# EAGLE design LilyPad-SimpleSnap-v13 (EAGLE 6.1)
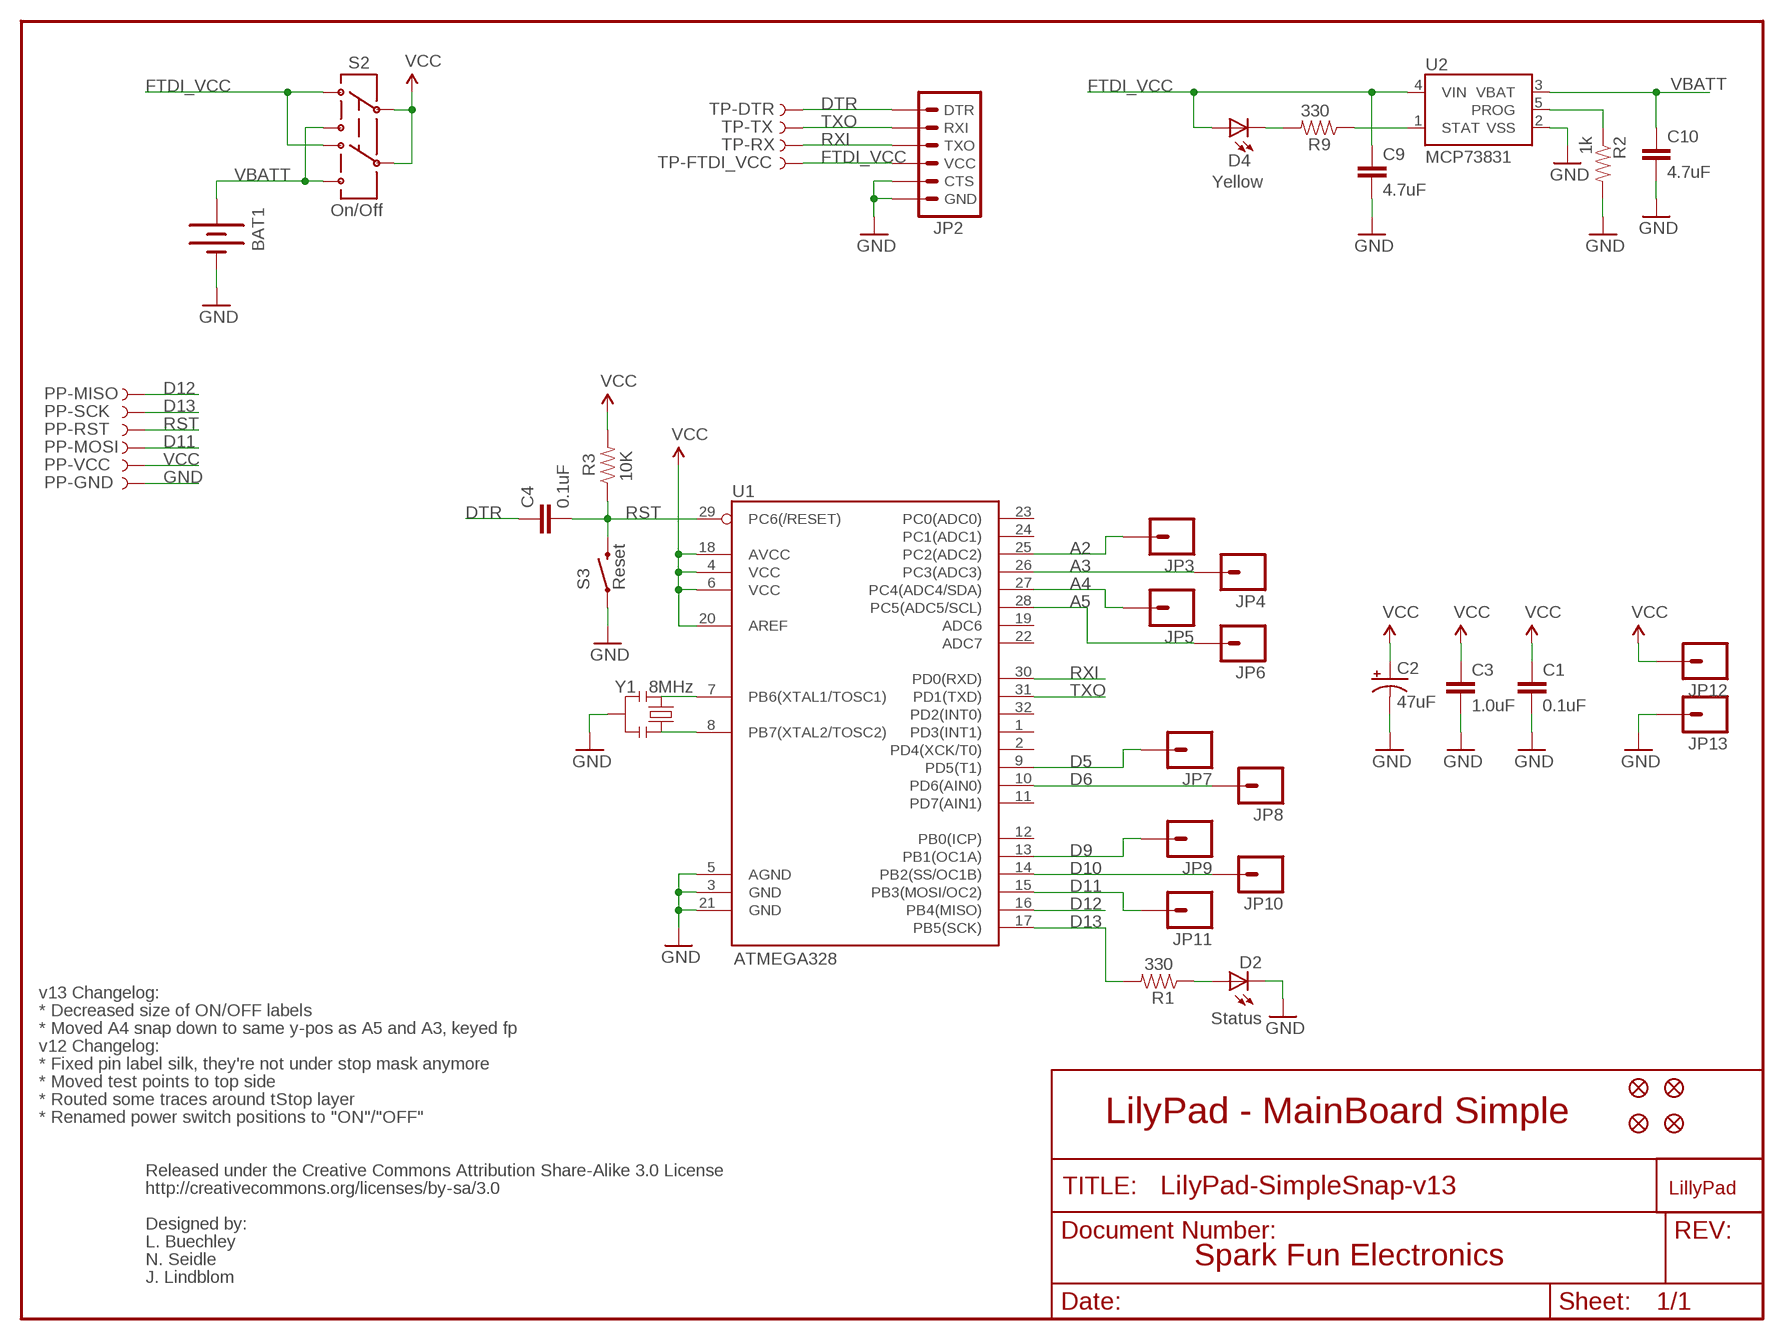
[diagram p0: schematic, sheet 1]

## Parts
BAT1  BATTERY110-TABS  [LIPO-110-TABS]
C1  0.1uF  CAP0402-CAP  [0402-CAP]
C2  47uF  CAP_POL3528  [EIA3528]
C3  1.0uF  CAP0402-CAP  [0402-CAP]
C4  0.1uF  CAP0402-CAP  [0402-CAP]
C9  4.7uF  CAP0402-CAP  [0402-CAP]
C10  4.7uF  CAP0402-CAP  [0402-CAP]
D2  Status  LED0603  [LED-0603]
D4  Yellow  LED0603  [LED-0603]
JP1  FIDUCIALUFIDUCIAL  [MICRO-FIDUCIAL]
JP2  ARDUINO_SERIAL_PROGRAMSMD  [1X06-SMD]
JP3  M01SNAP-FEMALE_LARGE  M01SNAP-FEMALE  [SNAP-FEMALE]
JP4  M01SNAP-FEMALE_LARGE  M01SNAP-FEMALE  [SNAP-FEMALE]
JP5  M01SNAP-FEMALE_LARGE  M01SNAP-FEMALE  [SNAP-FEMALE]
JP6  M01SNAP-FEMALE_LARGE  M01SNAP-FEMALE  [SNAP-FEMALE]
JP7  M01SNAP-FEMALE_LARGE  M01SNAP-FEMALE  [SNAP-FEMALE]
JP8  M01SNAP-FEMALE_LARGE  M01SNAP-FEMALE  [SNAP-FEMALE]
JP9  M01SNAP-FEMALE_LARGE  M01SNAP-FEMALE  [SNAP-FEMALE]
JP10  M01SNAP-FEMALE_LARGE  M01SNAP-FEMALE  [SNAP-FEMALE]
JP11  M01SNAP-FEMALE_LARGE  M01SNAP-FEMALE  [SNAP-FEMALE]
JP12  M01SNAP-FEMALE_LARGE  M01SNAP-FEMALE  [SNAP-FEMALE]
JP13  M01SNAP-FEMALE_LARGE  M01SNAP-FEMALE  [SNAP-FEMALE]
JP14  FIDUCIALUFIDUCIAL  [MICRO-FIDUCIAL]
JP15  FIDUCIALUFIDUCIAL  [MICRO-FIDUCIAL]
JP16  FIDUCIALUFIDUCIAL  [MICRO-FIDUCIAL]
PP-GND  TEST-POINT3X5  [PAD.03X.05]
PP-MISO  TEST-POINT3X5  [PAD.03X.05]
PP-MOSI  TEST-POINT3X5  [PAD.03X.05]
PP-RST  TEST-POINT3X5  [PAD.03X.05]
PP-SCK  TEST-POINT3X5  [PAD.03X.05]
PP-VCC  TEST-POINT3X5  [PAD.03X.05]
R1  330  RESISTOR0402-RES  [0402-RES]
R2  1k  RESISTOR0402-RES  [0402-RES]
R3  10K  RESISTOR0402-RES  [0402-RES]
R9  330  RESISTOR0402-RES  [0402-RES]
S2  On/Off  AYZ0202  [AYZ0202]
S3  Reset  SWITCH-MOMENTARY-2SMD  [TACTILE_SWITCH_SMD]
TP-DTR  TEST-POINT3X5  [PAD.03X.05]
TP-FTDI_VCC  TEST-POINT3X5  [PAD.03X.05]
TP-RX  TEST-POINT3X5  [PAD.03X.05]
TP-TX  TEST-POINT3X5  [PAD.03X.05]
U1  ATMEGA328  ATMEGA168  [TQFP32-08]
U2  MCP73831  [SOT23-5]
U$2  LOGO-LPLP  [LOGO-LILYPAD]
Y1  8MHz  RESONATORSMD  [RESONATOR-SMD]

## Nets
A2: JP3.1 U1.25(PC2(ADC2))
A3: JP4.1 U1.26(PC3(ADC3))
A4: JP5.1 U1.27(PC4(ADC4/SDA))
A5: JP6.1 U1.28(PC5(ADC5/SCL))
D5: JP7.1 U1.9(PD5(T1))
D6: JP8.1 U1.10(PD6(AIN0))
D9: JP9.1 U1.13(PB1(OC1A))
D10: JP10.1 U1.14(PB2(SS/OC1B))
D11: JP11.1 PP-MOSI.P$1 U1.15(PB3(MOSI/OC2))
D12: PP-MISO.P$1 U1.16(PB4(MISO))
D13: PP-SCK.P$1 R1.2 U1.17(PB5(SCK))
DTR: C4.1 JP2.1(DTR) TP-DTR.P$1
FTDI_VCC: C9.1 D4.A JP2.4(VCC) S2.3 S2.6 TP-FTDI_VCC.P$1 U2.4(VIN)
GND [VCC]: BAT1.- C1.2 C2.C(-) C3.2 C9.2 C10.2 D2.C JP2.5(CTS) JP2.6(GND) JP13.1 PP-GND.P$1 R2.2 S3.1 U1.3(GND) U1.5(AGND) U1.21(GND) U2.2(VSS) Y1.2
N$1: U1.7(PB6(XTAL1/TOSC1)) Y1.1
N$2: D2.A R1.1
N$3: U1.8(PB7(XTAL2/TOSC2)) Y1.3
N$8: D4.C R9.2
PROG: R2.1 U2.5(PROG)
RST: C4.2 PP-RST.P$1 R3.1 S3.3 U1.29(PC6(/RESET))
RXI: JP2.3(TXO) TP-RX.P$1 U1.30(PD0(RXD))
STAT: R9.1 U2.1(STAT)
TXO: JP2.2(RXI) TP-TX.P$1 U1.31(PD1(TXD))
VBATT: BAT1.+ C10.1 S2.1 S2.4 U2.3(VBAT)
VCC [VCC]: C1.1 C2.A(+) C3.1 JP12.1 PP-VCC.P$1 R3.2 S2.2 S2.5 U1.4(VCC) U1.6(VCC) U1.18(AVCC) U1.20(AREF)
Unconnected: U1.1(PD3(INT1)) U1.2(PD4(XCK/T0)) U1.11(PD7(AIN1)) U1.12(PB0(ICP)) U1.19(ADC6) U1.22(ADC7) U1.23(PC0(ADC0)) U1.24(PC1(ADC1)) U1.32(PD2(INT0))

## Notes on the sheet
- v13 Changelog:
- * Decreased size of ON/OFF labels
- * Moved A4 snap down to same y-pos as A5 and A3, keyed fp
- v12 Changelog:
- * Fixed pin label silk, they're not under stop mask anymore
- * Moved test points to top side
- * Routed some traces around tStop layer
- * Renamed power switch positions to "ON"/"OFF" | LilyPad - MainBoard Simple
- Released under the Creative Commons Attribution Share-Alike 3.0 License
- http://creativecommons.org/licenses/by-sa/3.0
- Designed by:
- L. Buechley
- N. Seidle | Spark Fun Electronics
- J. Lindblom

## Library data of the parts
BAT1 = SparkFun:BATTERY: Battery Holders
C1 C3 C4 C9 C10 = SparkFun:CAP: Capacitor
C2 = SparkFun:CAP_POL: Capacitor Polarized
D2 D4 = SparkFun:LED: LEDs
JP1 JP14-JP16 = SparkFun:FIDUCIAL: Fiducial Alignment Points
JP2 = SparkFun:ARDUINO_SERIAL_PROGRAM
JP3-JP13 = SparkFun:M01: Header 1
PP-GND PP-MISO PP-MOSI PP-RST PP-SCK PP-VCC TP-DTR TP-FTDI_VCC TP-RX TP-TX = SparkFun:TEST-POINT
R1-R3 R9 = SparkFun:RESISTOR: Resistor
S2 = SparkFun:AYZ0202: SPDT Slide Switch Simple SMD single-pull double-throw slide switch. Good for less than 350mA power switch, switching UARTs between devices, etc. Spark Fun Electronics SKU : COM-00597
S3 = SparkFun:SWITCH-MOMENTARY-2
U1 = SparkFun:ATMEGA168
U2 = SparkFun:MCP73831: Microchip's MCP73831 Miniature single cell, fully integrated Li-Ion, Li-polymer charge management controller http://ww1.microchip.com/downloads/en/DeviceDoc/21984a.pdf
U$2 = LilyPad-Wearables:LOGO-LP
Y1 = SparkFun:RESONATOR: Resonator Small SMD resonator. This is the itty bitty 10/20MHz resonators with built in caps. CSTCE10M0G55 and CSTCE20M0V53. Footprint has been reviewed closely but hasn't been tested yet.

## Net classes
0 Default: width 0.203 mm
1 VCC: width 0.254 mm

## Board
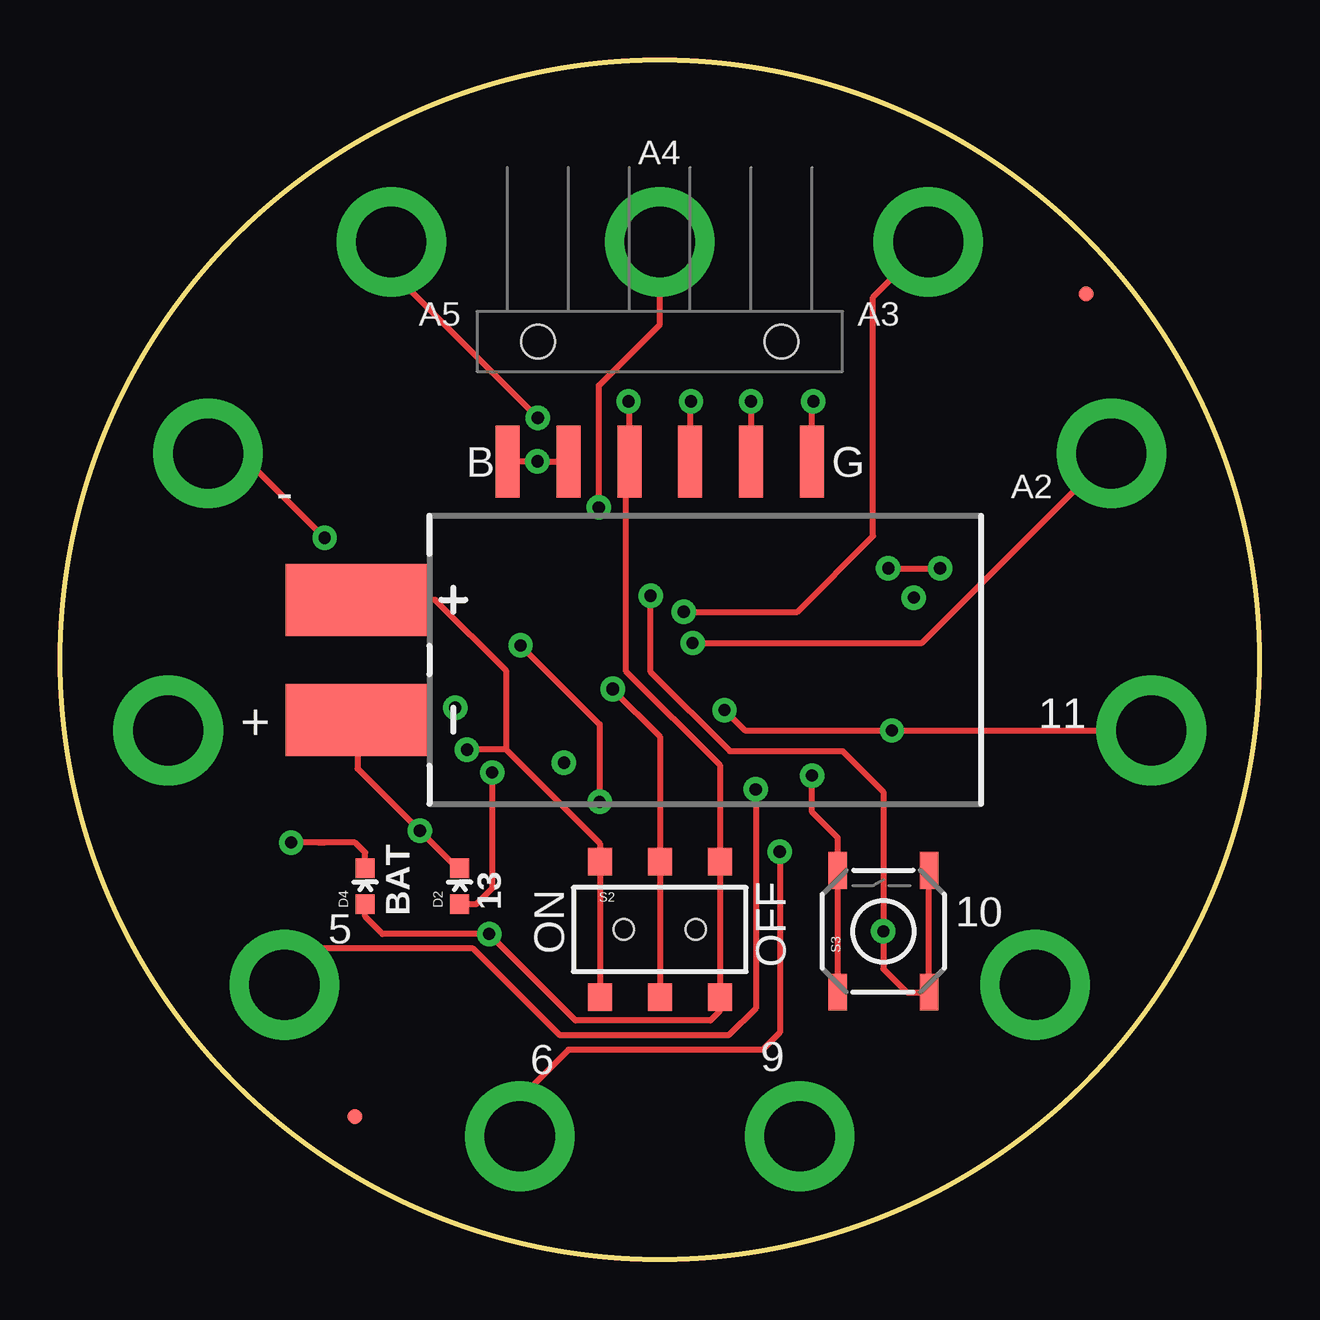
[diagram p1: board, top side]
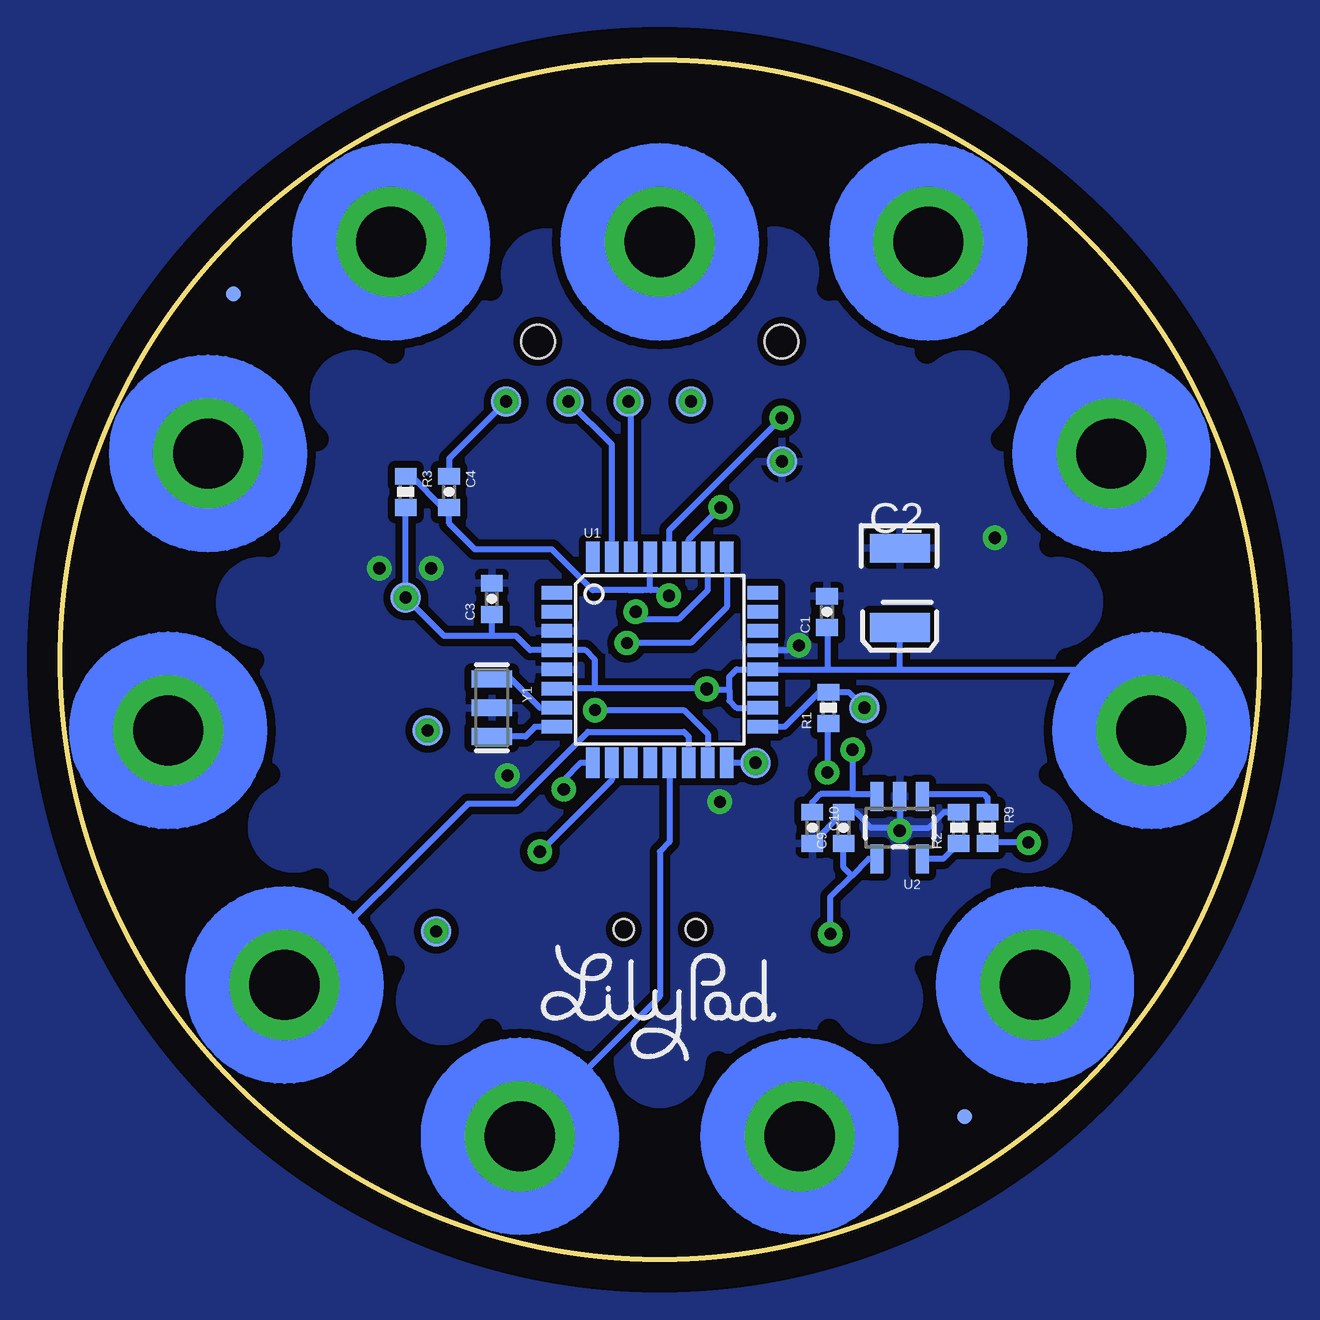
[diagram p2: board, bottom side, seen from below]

Size 50 x 50 mm. Coordinates in mm from the lower left corner, seen from the top.
Outline: circle at 25,25 radius 25
Copper layers (1*16): Top 0.035mm / dielectric 1.5mm / Bottom 0.035mm
Design rules: minimum track width 8mil, minimum drill 20mil, track to track 8mil, track to pad 8mil, pad to pad 8mil, via to via 8mil, smd to smd 8mil, copper to edge 8mil, drill to drill 8mil, minimum pad ring 12mil, minimum via ring 10mil, stop-mask expansion 4mil, vias tented up to drill 20mil, thermal gap 10mil
bRestrict: area 2.4,2.4 to 47.6,47.6; area 21,42.8 to 23.5,44; area 31.6,41.3 to 34.4,43; area 36.3,38.4 to 38.9,40.7; area 40,34.1 to 42,36.9; area 42.2,29.2 to 43.6,31.8; area 42.8,23.9 to 44,26.2; area 42.2,18.2 to 43.7,20.9; area 36.3,9.4 to 39,11.7; area 31.7,7 to 34.5,8.7; area 26.5,6 to 28.9,7.3; area 21.1,6 to 23.6,7.3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; 22 lines

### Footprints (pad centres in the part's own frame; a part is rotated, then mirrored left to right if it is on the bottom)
LIPO-110-TABS = smd 3 x 6: + 2.5,14.5; - -2.5,14.5
0402-CAP = smd 0.7 x 0.9: 1 -0.65,0; 2 0.65,0
EIA3528 = smd 1.2 x 2.5: A 1.65,0; C -1.65,0
LED-0603 = smd 0.8 x 0.8: A 0,-0.75; C 0,0.75
MICRO-FIDUCIAL = smd 0.635 x 0.635: 1 0,0
1X06-SMD = smd 1 x 3: 1 -6.35,5; 2 -3.81,5; 3 -1.27,5; 4 1.27,5; 5 3.81,5; 6 6.35,5 | hole 1.4: -5.08,0; 5.08,0
SNAP-FEMALE = drill 2.921 pad 4.572: 1 0,0
PAD.03X.05 = smd 1.27 x 1.27: P$1 0,0
0402-RES = smd 0.7 x 0.9: 1 -0.65,0; 2 0.65,0
AYZ0202 = smd 1 x 1.15: 1 -2.5,2.825; 2 0,2.825; 3 2.5,2.825; 4 -2.5,-2.825; 5 0,-2.825; 6 2.5,-2.825 | hole 0.85: 1.5,0; -1.5,0
TACTILE_SWITCH_SMD = smd 1.524 x 0.762: 1 -2.54,1.905; 2 2.54,1.905; 3 -2.54,-1.905; 4 2.54,-1.905
TQFP32-08 = smd 1.27 x 0.559: 1 -4.293,2.8; 2 -4.293,2; 3 -4.293,1.2; 4 -4.293,0.4; 5 -4.293,-0.4; 6 -4.293,-1.2; 7 -4.293,-2; 8 -4.293,-2.8; 17 4.293,-2.8; 18 4.293,-2; 19 4.293,-1.2; 20 4.293,-0.4; 21 4.293,0.4; 22 4.293,1.2; 23 4.293,2; 24 4.293,2.8 | smd 0.559 x 1.27: 9 -2.8,-4.293; 10 -2,-4.293; 11 -1.2,-4.293; 12 -0.4,-4.293; 13 0.4,-4.293; 14 1.2,-4.293; 15 2,-4.293; 16 2.8,-4.293; 25 2.8,4.293; 26 2,4.293; 27 1.2,4.293; 28 0.4,4.293; 29 -0.4,4.293; 30 -1.2,4.293; 31 -2,4.293; 32 -2.8,4.293
SOT23-5 = smd 0.55 x 1.2: 1 -0.95,-1.3; 2 0,-1.3; 3 0.95,-1.3; 4 0.95,1.3; 5 -0.95,1.3
RESONATOR-SMD = smd 0.7 x 1.7: 1 -1.2,0; 2 0,0; 3 1.2,0

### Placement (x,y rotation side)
BAT1  26.91,25 90 top
C1  18.03,27 90 bottom
C2  15,28 270 bottom
C3  32,27.54 90 bottom
C4  33.78,32 270 bottom
C9  17.34,18 90 bottom
C10  18.64,18 270 bottom
D2  16.66,15.56 0 top
D4  12.72,15.56 0 top
JP1  42.78,40.24 0 top
JP2  25,38.27 180 top
JP3  43.83,33.6 0 bottom
JP4  36.19,42.41 0 bottom
JP5  25,42.41 0 bottom
JP6  13.81,42.41 0 bottom
JP7  9.36,11.44 0 bottom
JP8  19.17,5.14 0 bottom
JP9  30.83,5.14 0 bottom
JP10  40.64,11.44 0 bottom
JP11  45.49,22.05 0 bottom
JP12  4.51,22.05 0 bottom
JP13  6.17,33.6 0 bottom
JP14  12.3,5.95 0 top
JP15  12.3,5.95 0 bottom
JP16  42.78,40.24 0 bottom
PP-GND  19.9,33.27 0 bottom
PP-MISO  21.01,20.71 180 bottom
PP-MOSI  34.68,22.05 0 bottom
PP-RST  34.32,13.68 0 bottom
PP-SCK  16.47,23 180 bottom
PP-VCC  35.59,27.59 0 bottom
R1  17.97,23 90 bottom
R2  12.54,18 90 bottom
R3  35.59,32 270 bottom
R9  11.34,18 270 bottom
S2  25,13.76 0 top
S3  34.32,13.68 90 top
TP-DTR  31.4,35.77 0 bottom
TP-FTDI_VCC  23.7,35.77 0 bottom
TP-RX  26.3,35.77 0 bottom
TP-TX  28.8,35.77 90 bottom
U1  25,25 0 bottom
U2  15,18 180 bottom
U$2  25,11.03 0 bottom
Y1  32,23 270 bottom

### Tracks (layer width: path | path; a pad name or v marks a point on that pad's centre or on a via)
A2  (via drill 0.51)
  Top 0.254: JP3.1 35.93,25.7 v26.37,25.7
  Bottom 0.254: v26.37,25.7 23.7,25.7 22.2,27.2 U1.25
A3  (via drill 0.51)
  Top 0.254: v26,27 30.73,27 33.89,30.16 33.89,40.11 JP4.1
  Bottom 0.254: U1.26 23,27.9 24.2,26.7 25.7,26.7 v26,27
A4  (via drill 0.51)
  Top 0.254: v22.46,31.35 22.46,36.43 25,38.97 JP5.1
  Bottom 0.254: U1.27 23.8,30.01 v22.46,31.35
A5  (via drill 0.51)
  Top 0.254: v19.92,35.08 13.81,41.19 JP6.1
  Bottom 0.254: U1.28 24.6,30.4 v19.92,35.08
D5  (via drill 0.51)
  Top 0.254: v29,19.6 29,10.48 27.87,9.35 20.84,9.35 17.23,12.96 10.87,12.96 JP7.1
  Bottom 0.254: U1.9 28.29,20.71 29,20 v29,19.6
D6  (via drill 0.51)
  Top 0.254: v30,17 30,9.46 29.28,8.74 21.19,8.74 19.17,6.72 JP8.1
  Bottom 0.254: U1.10 27,20 v30,17
D9
  Bottom 0.254: U1.13 24.6,17.4 25,17 25,10.97 JP9.1
D10
  Bottom 0.254: U1.14 23.8,21.8 24,22 28,22 31,19 33,19 40.56,11.44 JP10.1
D11  (via drill 0.51)
  Top 0.254: v27.7,22.9 28.55,22.05 PP-MOSI.P$1 JP11.1
  Bottom 0.254: U1.15 23,21.9 24,22.9 v27.7,22.9
  other vias: 34.68,22.05
D12  (via drill 0.51)
  Bottom 0.254: PP-MISO.P$1 U1.16
  other vias: 21.01,20.71
D13  (via drill 0.51)
  Bottom 0.254: U1.17 19.8,22.2 18.35,23.65 R1.2 17.12,23.65 PP-SCK.P$1
  other vias: 16.47,23
DTR  (via drill 0.51)
  Top 0.254: JP2.1 31.35,35.72 TP-DTR.P$1
  Bottom 0.254: C4.1 33.78,33.39 TP-DTR.P$1
  other vias: 31.4,35.77
FTDI_VCC  (via drill 0.51)
  Top 0.254: 23.73,33 JP2.4 | 23.73,33 23.6,32.87 23.6,24.51 27.5,20.61 S2.3 S2.6 27.5,10.36 27.11,9.97 21.49,9.97 v17.89,13.57 13.44,13.57 12.72,14.29 D4.A | 23.73,33 23.73,35.74 TP-FTDI_VCC.P$1
  Bottom 0.254: U2.4 16.3,16.7 17,16 | C9.1 17.34,16.34 17,16 | v17.89,13.57 17.89,15.11 17,16
  other vias: 23.7,35.77
GND  (via drill 0.51)
  Top 0.254: JP2.6 PP-GND.P$1 JP2.5 | v34.52,28.81 v36.68,28.81 | v31.35,20.17 31.35,18.65 32.41,17.59 S3.1 | D2.C 16.56,16.31 v15,17.87 12.4,20.47 BAT1.- | JP13.1 7.51,33.6 v11.03,30.08 | v22.49,19.08 22.49,22.31 v19.2,25.6
  Bottom 0.254: R2.2 13.15,18.65 13.8,18 14.97,18 | C10.2 C9.2 16.85,18.65 16.2,18 14.97,18 | v19.2,25.6 19.4,25.4 U1.21 | U2.2 15,18.03 14.97,18
  other vias: 19.9,33.27
  pour Bottom (isolate 0.305): -3.54,53.54 53.54,53.54 53.54,-3.54 -3.54,-3.54
N$1
  Bottom 0.254: U1.7 30,23 31.2,24.2 Y1.1
N$2  (via drill 0.51)
  Top 0.254: D2.A 17.35,14.81 18.02,15.47 v18.02,20.3
  Bottom 0.254: v18.02,20.3 18.02,22.3 R1.1
N$3
  Bottom 0.254: U1.8 30.2,22.2 30.6,21.8 Y1.3
N$8  (via drill 0.51)
  Top 0.254: 10.78,17.38 v9.63,17.38 | 10.78,17.38 11.03,17.38 | D4.C 12.72,16.96 12.3,17.38 10.78,17.38
  Bottom 0.254: v9.63,17.38 11.31,17.38 R9.2
PROG
  Bottom 0.254: R2.1 13.19,16.7 U2.5
RST  (via drill 0.51)
  Top 0.254: v24.62,27.67 24.62,24.49 27.92,21.19 32.62,21.19 34.32,19.49 PP-RST.P$1 34.32,12.12 35.3,11.14 S3.3 36.23,16.29
  Bottom 0.254: R3.1 35.35,32.65 34.05,31.35 C4.2 33.78,30.68 32.7,29.6 29.5,29.6 27.8,27.9 26.27,27.9 | 26.27,27.9 25.7,27.9 | v24.62,27.67 24.87,27.67 25.1,27.9 25.38,27.9 | 25.38,27.9 26.27,27.9 | U1.29 25.4,27.92 25.38,27.9
  other vias: 34.32,13.68
RXI  (via drill 0.51)
  Top 0.254: JP2.3 26.27,35.74 TP-RX.P$1
  Bottom 0.254: U1.30 26.2,35.67 TP-RX.P$1
  other vias: 26.3,35.77
STAT
  Bottom 0.254: R9.1 11.34,19.24 11.5,19.4 13.95,19.4 U2.1
TXO  (via drill 0.51)
  Top 0.254: JP2.2 TP-TX.P$1
  Bottom 0.254: U1.31 27,33.97 TP-TX.P$1
  other vias: 28.8,35.77
VBATT  (via drill 0.51)
  Top 0.254: S2.4 S2.1 22.5,17.34 18.59,21.25 | 18.59,21.25 18.59,24.56 15.64,27.5 BAT1.+ | 18.59,21.25 v16.97,21.25
  Bottom 0.254: C10.1 18.64,19.06 18.3,19.4 17,19.4 | 17,19.4 16.05,19.4 U2.3 | v16.97,21.25 16.97,19.43 17,19.4
VCC  (via drill 0.51)
  Top 0.254: S2.5 S2.2 25,21.8 v23.04,23.76 v23.04,23.8
  Bottom 0.254: 18,24.6 U1.20 21.8,24.6 22.1,24.3 22.1,23.73 | 18,24.6 15,24.6 | 15,24.6 C2.A | C1.1 18,26.32 18,24.6 | 22.1,23.73 22.1,23.3 21.8,23 U1.18 | 27.7,23.8 U1.6 | 27.7,23.8 27.7,25 28.1,25.4 U1.4 30.4,25.4 31,26 32,26 | R3.2 PP-VCC.P$1 34,26 32,26 | 32,26 C3.1 | v23.04,23.8 27.7,23.8 | v23.04,23.76 22.13,23.76 22.1,23.73 | 15,24.6 7.06,24.6 JP12.1
  other vias: 35.59,27.59

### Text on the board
tPlace: A4 | A5 | A3 | B | G | A2 | - | + | 11 | 13 | BAT | 10 | 5 | ON | OFF | 6 | 9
